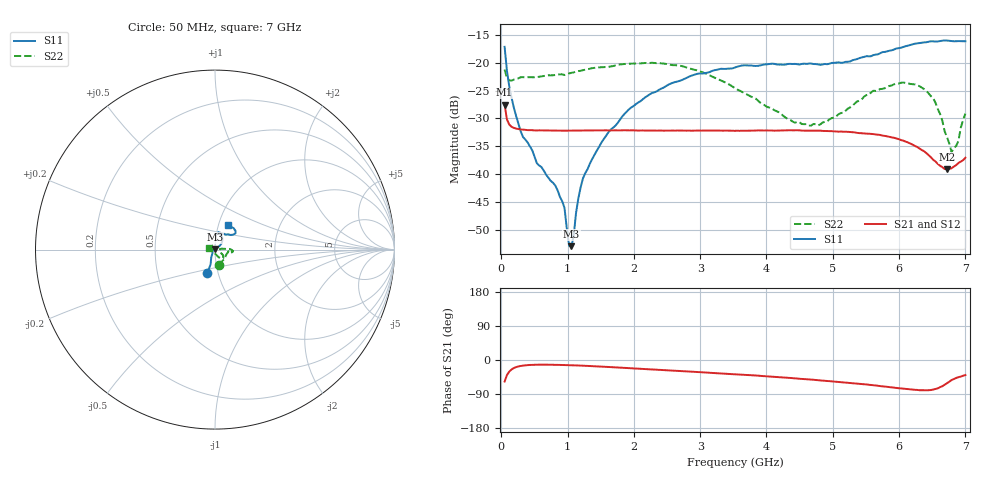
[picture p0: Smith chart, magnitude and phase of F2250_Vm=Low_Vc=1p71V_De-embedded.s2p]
! Integrated Device Technology
! Corporate Headquarters
! 6024 Silver Creek Valley Road
! San Jose, CA 95138  USA
! Phone:  1-408-284-8200
! Toll Free:  1-800-223-1366
! Webpage:  http://www.idt.com/
! Timing and RF Division
! 515 Groton Road, Suite 102
! Westford, MA 01886-6024
! Device:  F2250
! Description: Voltage Variable RF Attenuator
! Frequency:  50.0 -  6000.00 MHz
! Package:  3x3 mm Thin QFN Plastic Package: 16 pin
! Ports:  2 RF, 3 DC
!  Pin  1  = GND
!  Pin  2  = NC
!  Pin  3  = RF1  = Port 1
!  Pin  4  = NC
!  Pin  5  = GND
!  Pin  6  = GND
!  Pin  7  = GND
!  Pin  8  = GND
!  Pin  9  = NC
!  Pin 10  = RF2  = Port 2
!  Pin 11  = NC
!  Pin 12  = GND
!  Pin 13  = GND
!  Pin 14  = VCNTRL
!  Pin 15  = VDD
!  Pin 16  = VMODE
! Vcntrl:  1.710 Volts
! Vmode:  +0.000 Volts
! Vdd:  +3.30  Volts
! Current:  1.187 mA
! Data:  The device was measured on a the F2250 evaluation board which has
!  individual transmission lines to the RF pins.  Data was collected
!  using a calibrated network analyzer.  The evaluation board was
!  de-embedded using a TRL calibration technique.
!  The reference plane is the edge of the package pin.
! Misc:  SN 10
!  Action Tracker AT0258
! Date Measured:  2014-11-26
! Date:  2015-10-15  MJV
! Note:
!  Integrated Device Technology supplies this data as a sample of measured
!  data at the package pin for this product.  Your particular data for this
!  product may vary.
!  Data was taken at 25 degrees C.
!  Integrated Device Technology reserves the right to change this data at anytime.
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# GHz S dB R 50
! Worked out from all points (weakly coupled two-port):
!   201 points, 50 MHz to 7 GHz, reference 50 ohm
!   highest |S21| = -27.53 dB at 50 MHz (marker M1); lowest = -39.1 dB at 6.722 GHz (marker M2)
!   lowest |S11| = -52.9 dB at 1.058 GHz (marker M3), VSWR 1.00, Z = 49.9 + j0.212 ohm
!   |S11| at or under -10 dB: start of sweep to end of sweep
!   |S22| runs from -36.0 to -20.0 dB; largest |S21 - S12| = 0.00011
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0.05  -17.16 -108.0  -27.53 -56.8  -27.51 -56.7  -21.22 -76.1
0.1195  -24.20 -110.8  -31.08 -30.6  -31.06 -30.6  -23.15 -28.0
0.29325  -32.32 -125.7  -31.98 -15.7  -31.94 -15.7  -22.61 -12.6
0.5365  -38.02 -153.1  -32.15 -12.4  -32.13 -12.4  -22.59 -7.9
0.84925  -42.89 171.0  -32.18 -12.8  -32.17 -12.8  -22.13 -9.6
0.9535  -46.04 171.3  -32.20 -13.3  -32.19 -13.3  -22.21 -9.9
1.023  -52.81 138.0  -32.18 -13.6  -32.19 -13.6  -21.93 -9.5
1.05775  -52.90 110.0  -32.18 -13.8  -32.18 -13.8  -21.85 -9.4
1.162  -44.34 48.5  -32.16 -14.5  -32.15 -14.5  -21.50 -10.5
1.2315  -40.75 39.2  -32.15 -15.0  -32.16 -15.0  -21.34 -11.0
1.6485  -32.01 40.1  -32.15 -18.7  -32.14 -18.7  -20.69 -9.1
2.37825  -24.87 46.5  -32.16 -25.9  -32.15 -25.9  -20.06 -4.8
3.525  -20.86 72.1  -32.22 -37.7  -32.20 -37.7  -24.57 3.6
4.4285  -20.22 76.4  -32.12 -48.4  -32.11 -48.5  -30.75 3.1
4.7065  -20.23 72.1  -32.17 -52.2  -32.17 -52.2  -30.99 -7.6
5.85325  -17.85 40.2  -33.29 -71.5  -33.29 -71.5  -24.17 -41.3
6.40925  -16.33 41.6  -36.20 -79.8  -36.22 -79.8  -25.06 -56.6
6.54825  -16.21 44.9  -37.71 -76.5  -37.73 -76.5  -27.17 -66.0
6.722  -16.03 49.9  -39.09 -61.2  -39.11 -61.0  -33.34 -95.3
6.7915  -16.12 52.1  -38.93 -52.9  -38.92 -52.7  -36.03 -125.9
6.89575  -16.13 56.9  -37.98 -45.2  -37.97 -45.2  -33.99 -175.9
7  -16.16 63.0  -37.04 -39.7  -37.03 -39.6  -29.12 161.9
